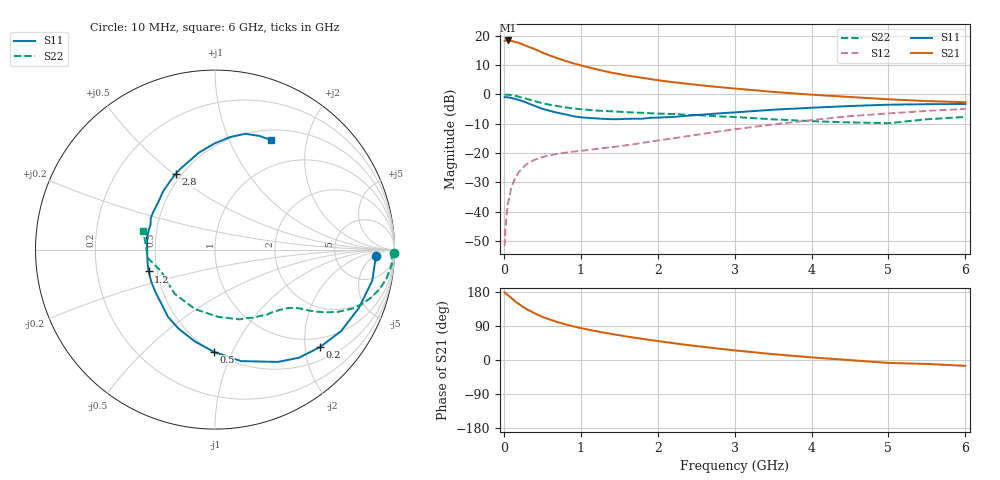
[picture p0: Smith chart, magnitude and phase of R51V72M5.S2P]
! SIEMENS Small Signal Semiconductors
! BFR183
! Si NPN RF Bipolar Junction Transistor in SOT23
! VCE = 1.75 V  IC = 2.5 mA
! Common Emitter S-Parameters:  May  1996
# GHz  S  MA  R  50
!  f  S11  S21  S12  S22
! GHz  MAG  ANG  MAG  ANG  MAG  ANG  MAG  ANG
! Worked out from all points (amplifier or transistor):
!   36 points, 10 MHz to 6 GHz, reference 50 ohm
!   highest |S21| = 18.4 dB at 50 MHz (marker M1)
!   |S21| within 3 dB of that: start of sweep to 404.5 MHz
!   unconditionally stable (mu >= 1): 1.289 GHz to 2.825 GHz
!   at 250 MHz: K = 0.26, MSG = 20.9 dB, |S12| = -24.9 dB
!   at 1.4 GHz: K = 1.04, MAG = 11.4 dB, |S12| = -18.0 dB
!   at 6 GHz: K = 0.91, MSG = 1.2 dB, |S12| = -5.0 dB
!   S11 on the Smith chart (normalised r, x): 10 MHz: 16, -6; 200 MHz: 0.78, -2.33; 500 MHz: 0.51, -0.85; 1.2 GHz: 0.45, -0.13; 2.8 GHz: 0.46, +0.51; 6 GHz: 0.63, +1.44
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0.01  0.8963 -2.3  8.228 178.6  0.0026 89.4  0.9952 -1.0
0.02  0.8941 -4.6  8.152 176.5  0.0051 89.0  0.9853 -1.9
0.05  0.8933 -11.1  8.282 171.4  0.0132 82.4  0.9889 -4.8
0.1  0.8652 -22.1  8.117 163.2  0.0266 78.3  0.9697 -9.4
0.15  0.8367 -32.8  7.77 154.3  0.0382 72.0  0.9433 -13.5
0.2  0.7987 -42.8  7.511 147.0  0.0486 67.3  0.9077 -17.3
0.25  0.7625 -52.2  7.043 140.0  0.057 62.8  0.8715 -20.5
0.3  0.7175 -60.7  6.607 133.8  0.0655 59.5  0.8366 -23.0
0.4  0.6379 -76.9  5.899 123.3  0.077 53.7  0.7674 -26.9
0.5  0.5688 -90.8  5.152 113.8  0.0848 49.8  0.7074 -29.6
0.6  0.5233 -102.5  4.574 106.7  0.0919 47.2  0.6637 -31.4
0.8  0.4575 -124.9  3.71 94.2  0.1016 44.5  0.6016 -33.8
0.9  0.4238 -135.0  3.392 88.9  0.1059 44.7  0.577 -34.7
1.1  0.3975 -153.2  2.891 80.1  0.1135 45.4  0.5441 -36.7
1.2  0.3896 -161.8  2.685 75.9  0.1172 46.0  0.5313 -37.7
1.6  0.3836 170.5  2.089 61.8  0.1365 48.9  0.4979 -42.2
2.2  0.4126 139.9  1.613 44.5  0.1778 52.7  0.4634 -51.7
2.8  0.4753 117.5  1.329 29.9  0.2343 52.1  0.4211 -64.9
3.5  0.5481 99.3  1.102 15.4  0.3069 46.8  0.3754 -87.1
4.5  0.6335 82.2  0.903 -0.4  0.4261 34.8  0.3334 -132.5
5.5  0.6799 68.6  0.768 -10.4  0.5232 20.9  0.3766 -172.9
6  0.6857 63.0  0.736 -15.4  0.5647 12.1  0.4127 165.3
